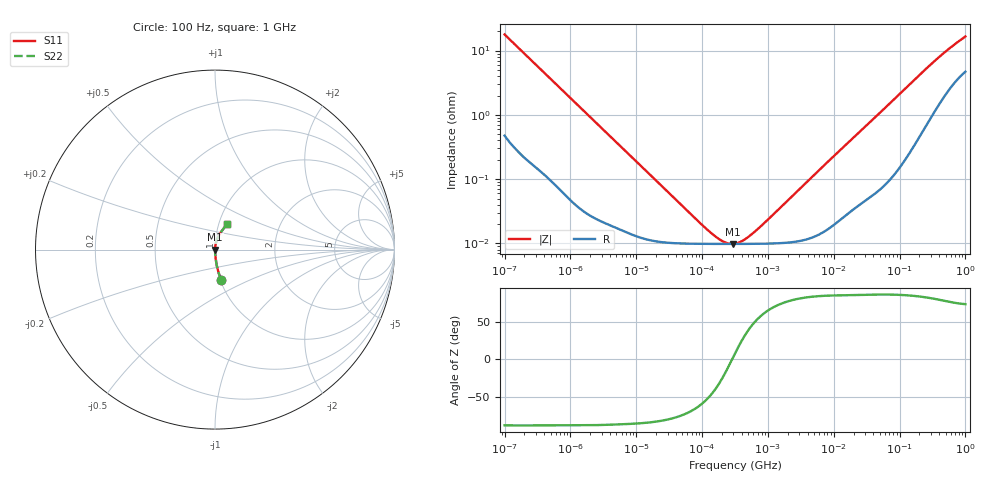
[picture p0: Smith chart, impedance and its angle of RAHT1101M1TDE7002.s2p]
! RAHT1101M1TDE7002  S-PARAMETER MODEL  (AEC-Q200 qualified)
! Model Generated by ELNA Corporation (http://www.ty-top.com)
! Version 1.0
! ELNA Control No. 240229
! Copyright (c) 2024 ELNA CO.,LTD. All Rights Reserved.
! Products Name : CONDUCTIVE POLYMER HYBRID ALUMINUM ELECTROLYTIC CAPACITORS
! Characteristics :
!  Capacitance  :  100uF  ,  Rated voltage  :  25V
!  Operating Temp. Range  :  -55 to +105 degC  ,  Endurance  :  5000hr at 105 degC
!  Dimension D  :  :  6.3mm  ,  Dimension L  :  7.7mm
! Frequency Range : 100Hz - 1GHz
! External Node Assignments :
!  1  o---| |---o  2
# MHz S RI R 50
!Freq[MHz].  S11 Real  S11 Imag  S21 Real  S21 Imag  S12 Real  S12 Imag  S22 Real  S22 Imag
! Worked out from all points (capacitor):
!   401 points, 100 Hz to 1 GHz, reference 50 ohm
!   read as one part in series: C = 89.3 uF near 108 Hz
!   lowest |Z| = 9.83 mohm at 291.7 kHz (marker M1)
!   series resonance near 286.6 kHz, so ESL is about 3.5 nH
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0.0001  0.035 -0.171  0.965 0.171  0.965 0.171  0.035 -0.171
0.000113  0.0281 -0.1528  0.9719 0.1528  0.9719 0.1528  0.0281 -0.1528
0.000183  0.0117 -0.0963  0.9883 0.0963  0.9883 0.0963  0.0117 -0.0963
0.000309  0.00483 -0.0578  0.9952 0.0578  0.9952 0.0578  0.00483 -0.0578
0.000613  0.00165 -0.0296  0.9983 0.0296  0.9983 0.0296  0.00165 -0.0296
0.001488  0.000483 -0.0123  0.9995 0.0123  0.9995 0.0123  0.000483 -0.0123
0.022131  0.000107 -0.000853  0.9999 0.000853  0.9999 0.000853  0.000107 -0.000853
0.083657  9.87e-05 -0.000208  0.9999 0.000208  0.9999 0.000208  9.87e-05 -0.000208
0.147062  9.83e-05 -9.54e-05  0.9999 9.54e-05  0.9999 9.54e-05  9.83e-05 -9.54e-05
0.179887  9.83e-05 -6.41e-05  0.9999 6.41e-05  0.9999 6.41e-05  9.83e-05 -6.41e-05
0.220039  9.83e-05 -3.55e-05  0.9999 3.55e-05  0.9999 3.55e-05  9.83e-05 -3.55e-05
0.291743  9.83e-05 2.37e-06  0.9999 -2.37e-06  0.9999 -2.37e-06  9.83e-05 2.37e-06
0.316228  9.83e-05 1.31e-05  0.9999 -1.31e-05  0.9999 -1.31e-05  9.83e-05 1.31e-05
0.356862  9.83e-05 2.94e-05  0.9999 -2.94e-05  0.9999 -2.94e-05  9.83e-05 2.94e-05
0.419276  9.83e-05 5.18e-05  0.9999 -5.18e-05  0.9999 -5.18e-05  9.83e-05 5.18e-05
0.627336  9.86e-05 0.000115  0.9999 -0.000115  0.9999 -0.000115  9.86e-05 0.000115
4.704354  0.000125 0.00108  0.9999 -0.00108  0.9999 -0.00108  0.000125 0.00108
69.9842  0.00118 0.0148  0.9988 -0.0148  0.9988 -0.0148  0.00118 0.0148
169.8244  0.00466 0.0352  0.9953 -0.0352  0.9953 -0.0352  0.00466 0.0352
365.1741  0.0175 0.0702  0.9825 -0.0702  0.9825 -0.0702  0.0175 0.0702
641.9482  0.0403 0.1073  0.9597 -0.1073  0.9597 -0.1073  0.0403 0.1073
1000  0.0663 0.1417  0.9337 -0.1417  0.9337 -0.1417  0.0663 0.1417
